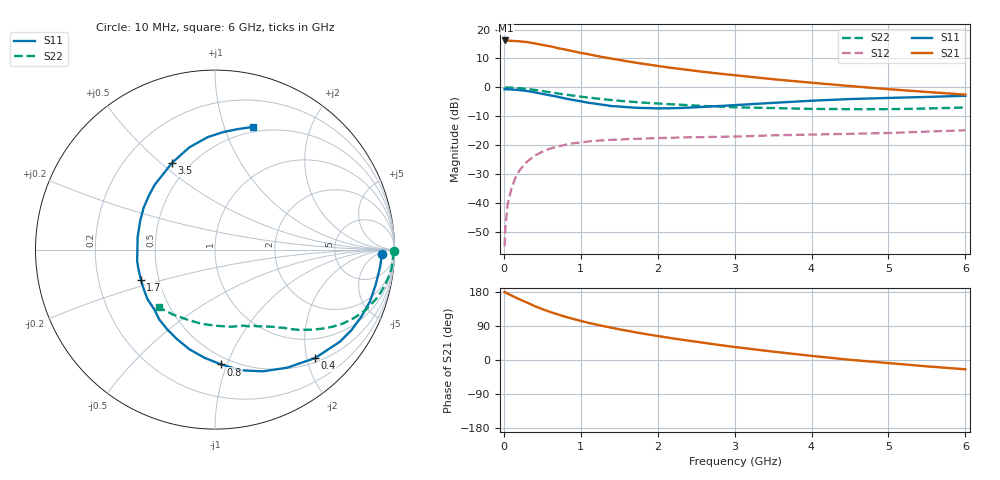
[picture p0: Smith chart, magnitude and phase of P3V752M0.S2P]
! SIEMENS Small Signal Semiconductors
! BFP181
! Si NPN RF Bipolar Junction Transistor in SOT143
! VCE = 0.75 V  IC = 2 mA
! Common Emitter S-Parameters:  March  1996
# GHz  S  MA  R  50
!  f  S11  S21  S12  S22
! GHz  MAG  ANG  MAG  ANG  MAG  ANG  MAG  ANG
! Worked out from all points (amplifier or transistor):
!   36 points, 10 MHz to 6 GHz, reference 50 ohm
!   highest |S21| = 16.2 dB at 20 MHz (marker M1)
!   |S21| within 3 dB of that: start of sweep to 770.3 MHz
!   unconditionally stable (mu >= 1): 2.186 GHz to end of sweep
!   at 250 MHz: K = 0.14, MSG = 21.5 dB, |S12| = -27.2 dB
!   at 1.4 GHz: K = 0.71, MSG = 14.0 dB, |S12| = -18.1 dB
!   at 6 GHz: K = 1.26, MAG = 3.1 dB, |S12| = -14.8 dB
!   S11 on the Smith chart (normalised r, x): 10 MHz: 25, -8; 400 MHz: 0.58, -2.15; 800 MHz: 0.44, -0.95; 1.7 GHz: 0.40, -0.17; 3.5 GHz: 0.40, +0.55; 6 GHz: 0.45, +1.25
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0.01  0.9293 -1.4  6.457 179.3  0.0018 85.5  0.9948 -0.5
0.02  0.9286 -2.6  6.468 178.7  0.0037 89.1  0.993 -1.2
0.05  0.9252 -5.9  6.439 175.1  0.0096 85.9  0.9922 -3.0
0.15  0.9105 -18.5  6.313 165.3  0.0272 78.4  0.979 -8.9
0.25  0.8827 -30.6  6.158 155.8  0.0437 71.6  0.9535 -14.5
0.3  0.8647 -36.4  6.065 151.7  0.0517 68.3  0.9383 -17.1
0.4  0.8221 -47.3  5.754 142.4  0.0656 62.0  0.9041 -21.9
0.5  0.7715 -58.5  5.416 134.3  0.0774 56.0  0.8643 -26.1
0.6  0.7285 -68.6  5.14 127.0  0.0874 51.0  0.8247 -29.9
0.7  0.6878 -77.9  4.772 120.4  0.0952 46.5  0.7855 -33.1
0.8  0.6406 -87.0  4.5 114.1  0.1017 42.5  0.7516 -35.7
0.9  0.6062 -95.4  4.215 108.5  0.108 39.1  0.7206 -38.0
1.1  0.5422 -112.9  3.74 98.0  0.116 33.5  0.6661 -42.1
1.4  0.4744 -135.6  3.137 85.2  0.1239 27.0  0.6037 -47.1
1.7  0.4457 -157.9  2.69 73.6  0.1287 22.9  0.559 -50.9
1.9  0.4386 -171.7  2.459 66.6  0.1316 20.4  0.5351 -53.5
2.2  0.4367 170.6  2.153 57.0  0.1349 17.9  0.5076 -57.5
2.8  0.4756 140.8  1.73 39.6  0.1401 14.2  0.4672 -66.2
3.5  0.5395 116.3  1.384 22.1  0.1481 11.0  0.4389 -78.4
4.5  0.6281 93.7  1.054 0.6  0.1575 6.9  0.4202 -100.1
5.5  0.6836 79.2  0.833 -16.8  0.172 4.8  0.4311 -123.0
6  0.7148 73.0  0.749 -24.5  0.1812 2.6  0.4492 -134.4
